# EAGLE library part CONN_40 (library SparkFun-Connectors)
Multi connection point. Often used as Generic Header-pin footprint for 0.1 inch spaced/style header connections On any of the 0.1 inch spaced packages, you can populate with these: Break Away Headers - Straight (PRT-00116) Break Away Male Headers - Right Angle (PRT-00553) Female Headers (PRT-00115) Break Away Headers - Machine Pin (PRT-00117) Break Away Female Headers - Swiss Machine Pin (PRT-00743) For SCREWTERMINALS and SPRING TERMINALS visit here: Screw Terimnals on SparkFun.com (5mm/3.5mm/2.54mm spacing) This device is also useful as a general connection point to wire up your design to another part of your project. Our various solder wires solder well into these plated through hole pads. Hook-Up Wire - Assortment (Stranded, 22 AWG) (PRT-11375) Hook-Up Wire - Assortment (Solid Core, 22 AWG) (PRT-11367) View the entire wire category on our website here Special notes: Molex polarized connector foot print use with SKU : PRT-08231 with associated crimp pins and housings. 1MM SMD Version SKU: PRT-10208 NOTES ON THE VARIANTS LOCK and LOCK_LONGPADS... This footprint was designed to help hold the alignment of a through-hole component (i.e. 6-pin header) while soldering it into place. You may notice that each hole has been shifted either up or down by 0.005 of an inch from it's more standard position (which is a perfectly straight line). This slight alteration caused the pins (the squares in the middle) to touch the edges of the holes. Because they are alternating, it causes a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
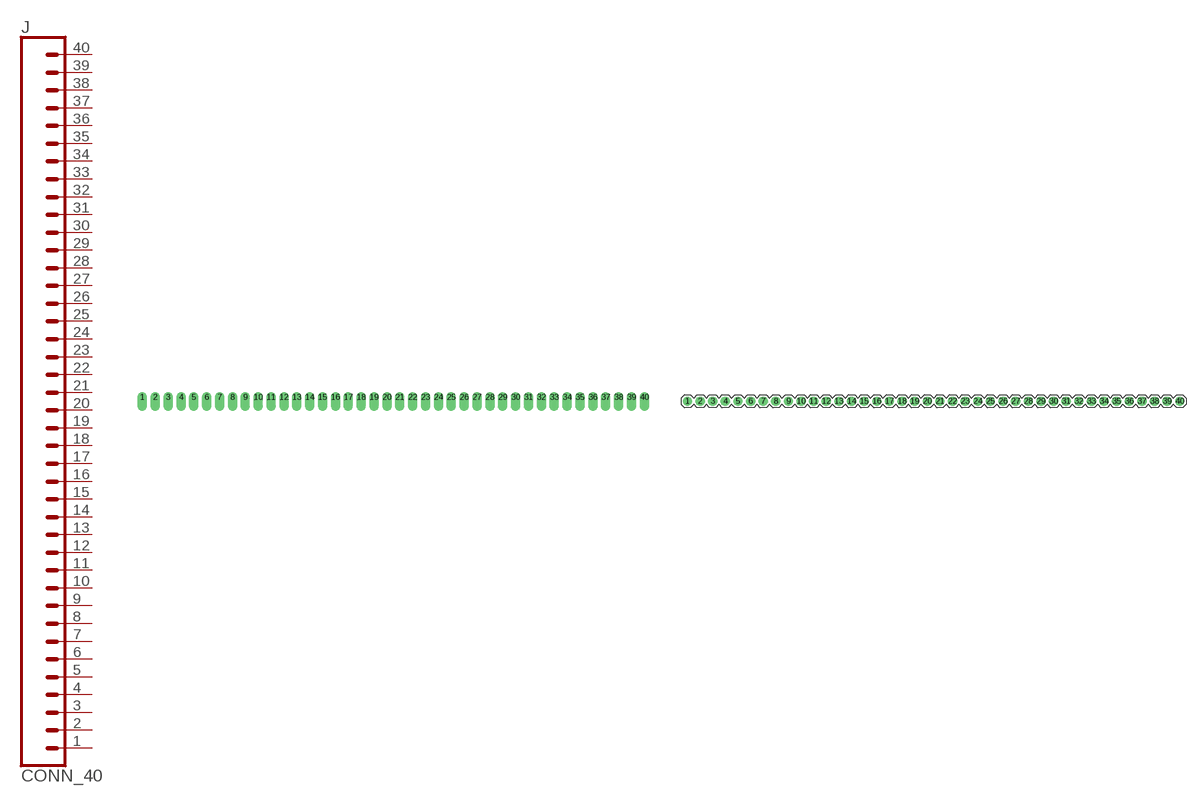
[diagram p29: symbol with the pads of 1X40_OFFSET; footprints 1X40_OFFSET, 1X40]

Designator prefix J

## CONN_40OFFSET  [1X40_OFFSET]
1  1  pas
2  2  pas
3  3  pas
4  4  pas
5  5  pas
6  6  pas
7  7  pas
8  8  pas
9  9  pas
10  10  pas
11  11  pas
12  12  pas
13  13  pas
14  14  pas
15  15  pas
16  16  pas
17  17  pas
18  18  pas
19  19  pas
20  20  pas
21  21  pas
22  22  pas
23  23  pas
24  24  pas
25  25  pas
26  26  pas
27  27  pas
28  28  pas
29  29  pas
30  30  pas
31  31  pas
32  32  pas
33  33  pas
34  34  pas
35  35  pas
36  36  pas
37  37  pas
38  38  pas
39  39  pas
40  40  pas

## CONN_40  [1X40]
Pads as for 1X40_OFFSET

## CONN_40-FPC (PROD_ID: CONN-14082)  [FPC05040-17204]
P$1  1  pas
P$2  2  pas
P$3  3  pas
P$4  4  pas
P$5  5  pas
P$6  6  pas
P$7  7  pas
P$8  8  pas
P$9  9  pas
P$10  10  pas
P$11  11  pas
P$12  12  pas
P$13  13  pas
P$14  14  pas
P$15  15  pas
P$16  16  pas
P$17  17  pas
P$18  18  pas
P$19  19  pas
P$20  20  pas
P$21  21  pas
P$22  22  pas
P$23  23  pas
P$24  24  pas
P$25  25  pas
P$26  26  pas
P$27  27  pas
P$28  28  pas
P$29  29  pas
P$30  30  pas
P$31  31  pas
P$32  32  pas
P$33  33  pas
P$34  34  pas
P$35  35  pas
P$36  36  pas
P$37  37  pas
P$38  38  pas
P$39  39  pas
P$40  40  pas

## Footprint 1X40_OFFSET (pad centres in mm)
Plated Through Hole -40 Pins Offset Long Pads + offset holes Specifications: Pin count:40 Pin pitch:0.1" Example device(s): CONN_40
drill 1.016 pad 1.88 offset: 1 0,0; 2 2.54,0; 3 5.08,0; 4 7.62,0; 5 10.16,0; 6 12.7,0; 7 15.24,0; 8 17.78,0; 9 20.32,0; 10 22.86,0; 11 25.4,0; 12 27.94,0; 13 30.48,0; 14 33.02,0; 15 35.56,0; 16 38.1,0; 17 40.64,0; 18 43.18,0; 19 45.72,0; 20 48.26,0; 21 50.8,0; 22 53.34,0; 23 55.88,0; 24 58.42,0; 25 60.96,0; 26 63.5,0; 27 66.04,0; 28 68.58,0; 29 71.12,0; 30 73.66,0; 31 76.2,0; 32 78.74,0; 33 81.28,0; 34 83.82,0; 35 86.36,0; 36 88.9,0; 37 91.44,0; 38 93.98,0; 39 96.52,0; 40 99.06,0

## Footprint 1X40 (pad centres in mm)
Plated Through Hole -40 Pins Specifications: Pin count:40 Pin pitch:0.1" Example device(s): CONN_40
drill 1.016 pad 1.88: 1 0,0; 2 2.54,0; 3 5.08,0; 4 7.62,0; 5 10.16,0; 6 12.7,0; 7 15.24,0; 8 17.78,0; 9 20.32,0; 10 22.86,0; 11 25.4,0; 12 27.94,0; 13 30.48,0; 14 33.02,0; 15 35.56,0; 16 38.1,0; 17 40.64,0; 18 43.18,0; 19 45.72,0; 20 48.26,0; 21 50.8,0; 22 53.34,0; 23 55.88,0; 24 58.42,0; 25 60.96,0; 26 63.5,0; 27 66.04,0; 28 68.58,0; 29 71.12,0; 30 73.66,0; 31 76.2,0; 32 78.74,0; 33 81.28,0; 34 83.82,0; 35 86.36,0; 36 88.9,0; 37 91.44,0; 38 93.98,0; 39 96.52,0; 40 99.06,0

## Footprint FPC05040-17204 (pad centres in mm)
This is a 40-pin FPC connector supplied by Atom. SparkFun SKU is CONN-14082
smd 0.3 x 1.2: P$1 -9.75,0.6; P$2 -9.25,0.6; P$3 -8.75,0.6; P$4 -8.25,0.6; P$5 -7.75,0.6; P$6 -7.25,0.6; P$7 -6.75,0.6; P$8 -6.25,0.6; P$9 -5.75,0.6; P$10 -5.25,0.6; P$11 -4.75,0.6; P$12 -4.25,0.6; P$13 -3.75,0.6; P$14 -3.25,0.6; P$15 -2.75,0.6; P$16 -2.25,0.6; P$17 -1.75,0.6; P$18 -1.25,0.6; P$19 -0.75,0.6; P$20 -0.25,0.6; P$21 0.25,0.6; P$22 0.75,0.6; P$23 1.25,0.6; P$24 1.75,0.6; P$25 2.25,0.6; P$26 2.75,0.6; P$27 3.25,0.6; P$28 3.75,0.6; P$29 4.25,0.6; P$30 4.75,0.6; P$31 5.25,0.6; P$32 5.75,0.6; P$33 6.25,0.6; P$34 6.75,0.6; P$35 7.25,0.6; P$36 7.75,0.6; P$37 8.25,0.6; P$38 8.75,0.6; P$39 9.25,0.6; P$40 9.75,0.6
